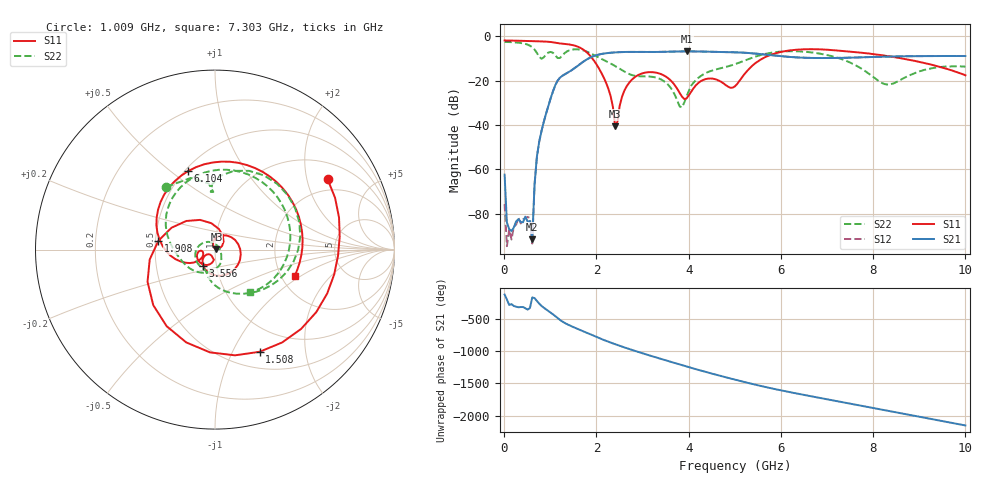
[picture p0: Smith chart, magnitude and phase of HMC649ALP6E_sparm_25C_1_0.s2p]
!Analog Devices Inc..
!GaAs MMIC 6-BIT DIGITAL PHASE SHIFTER, 3 - 6 GHz
!Filename: HMC649ALP6E_sparm_25C_1_0.s2p
!  :25C = 25degC
!  :_1_ = Sn1
!  :_0  = 0 state
!Device type:
!2 Port Calibration to sma connectors
!Phase Shifter:  0.000
!	Vss= -5V, Vdd= +5V , control Voltage = 0/ +5V
!Freq	S11	S11	S21	S21	S12	S12	S22	S22
! GHz	Mag dB	Degrees	Mag dB	Degrees	Mag dB	Degrees	Mag dB	Degrees
# GHZ S DB R 50.0
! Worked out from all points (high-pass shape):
!   201 points, 10 MHz to 10 GHz, reference 50 ohm
!   highest |S21| = -6.84 dB at 3.956 GHz (marker M1); lowest = -91.6 dB at 609.4 MHz (marker M2)
!   |S21| within 3 dB of the highest: 1.847 GHz to 6.749 GHz (4.902 GHz wide, 114 % of centre); 7.126 GHz to end of sweep
!   lowest |S11| = -40.7 dB at 2.408 GHz (marker M3), VSWR 1.02, Z = 50.8 + j0.396 ohm
!   |S11| at or under -10 dB: 1.911 GHz to 5.608 GHz (3.698 GHz wide, 98.4 % of centre); 8.614 GHz to end of sweep
!   |S22| runs from -32.1 to -2.6 dB; largest |S21 - S12| = 0.00074
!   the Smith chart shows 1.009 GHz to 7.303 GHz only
!   S11 on the Smith chart (normalised r, x): 1.009 GHz: 1.54, +2.68; 1.508 GHz: 0.69, -1.28; 1.908 GHz: 0.52, +0.06; 3.556 GHz: 0.86, -0.16; 6.104 GHz: 0.52, +0.58; 7.303 GHz: 2.35, -0.90
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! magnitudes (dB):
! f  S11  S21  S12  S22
! 10 MHz  -1.9  -62.5  -75.8  -2.6
! 59.95 MHz  -1.9  -84.0  -94.7  -2.6
! 609.4 MHz  -2.2  -91.6  -93.6  -5.0
! 759.2 MHz  -2.3  -47.7  -47.7  -9.2
! 1.009 GHz  -2.6  -28.0  -28.0  -7.1
! 1.508 GHz  -4.1  -14.7  -14.7  -6.0
! 1.708 GHz  -5.9  -11.6  -11.6  -6.4
! 1.908 GHz  -9.9  -9.2  -9.2  -8.1
! 2.258 GHz  -23.6  -7.6  -7.6  -11.8
! 2.408 GHz  -40.7  -7.3  -7.3  -13.5
! 2.707 GHz  -21.1  -7.1  -7.1  -17.0
! 3.357 GHz  -16.8  -7.1  -7.1  -19.1
! 3.556 GHz  -19.0  -7.0  -7.0  -21.9
! 3.806 GHz  -25.6  -6.9  -6.9  -31.7
! 3.956 GHz  -28.0  -6.8  -6.8  -27.1
! 4.356 GHz  -19.4  -7.0  -7.0  -16.8
! 5.005 GHz  -22.6  -7.3  -7.2  -12.6
! 6.104 GHz  -6.7  -9.2  -9.2  -6.8
! 6.703 GHz  -5.9  -9.8  -9.8  -7.4
! 7.303 GHz  -6.6  -9.8  -9.8  -10.2
! 8.352 GHz  -9.1  -9.2  -9.2  -21.8
! 10 GHz  -17.6  -9.0  -8.9  -13.7
